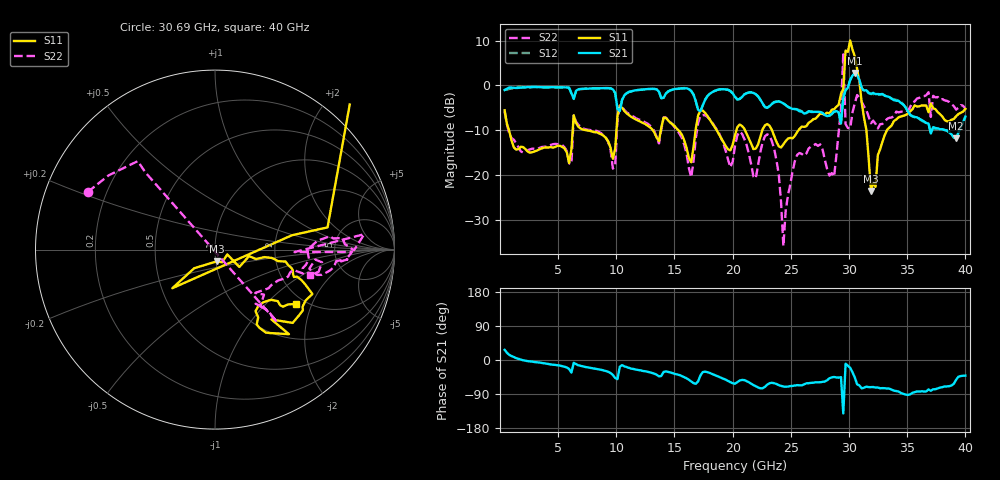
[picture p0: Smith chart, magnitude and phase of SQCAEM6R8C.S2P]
! Network Analyzer HP8722ES.07.66: Jul 25, 2000 Serial No. US39175408
! 26 Oct 2004  15:42:35
! Frequency  S11  S21  S12  S22
# HZ  S  DB R  50
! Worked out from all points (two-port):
!   201 points, 400 MHz to 40 GHz, reference 50 ohm
!   highest |S21| = 2.74 dB at 30.5 GHz (marker M1); lowest = -11.8 dB at 39.21 GHz (marker M2)
!   |S21| within 3 dB of the highest: 29.93 GHz to 31.05 GHz (1.12 GHz wide, 3.67 % of centre)
!   lowest |S11| = -23.6 dB at 31.88 GHz (marker M3), VSWR 1.14, Z = 50.6 - j6.64 ohm
!   |S11| at or under -10 dB: 771.5 MHz to 6.254 GHz (5.483 GHz wide, 156 % of centre); 7.361 GHz to 10.02 GHz (2.654 GHz wide, 30.6 % of centre); 23.38 GHz to 25.67 GHz (2.294 GHz wide, 9.35 % of centre)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
!   |S22| runs from -35.9 to 6.9 dB; largest |S21 - S12| = 0.17
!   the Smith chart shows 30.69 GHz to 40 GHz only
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4e8  -5.57 -66.2  -1.05 26.9  -1.00 30.4  -5.82 -58.9
7.132e9  -9.89 -101.3  -0.78 -17.1  -0.81 -17.5  -9.58 -112.5
1.3666e10  -12.44 -99.6  -1.43 -43.3  -1.44 -43.1  -12.98 -104.7
2.02e10  -11.18 -75.4  -2.60 -62.6  -2.54 -61.8  -13.53 -73.5
2.317e10  -9.04 -90.7  -4.67 -61.2  -4.63 -60.7  -11.22 -105.8
2.4358e10  -13.17 -70.4  -4.04 -70.1  -4.06 -69.2  -35.91 -91.4
2.5348e10  -11.27 -55.1  -5.31 -67.2  -5.27 -67.7  -16.91 -16.2
2.6932e10  -7.56 -54.4  -5.93 -59.9  -5.94 -59.7  -13.42 -31.8
2.8714e10  -5.36 -45.3  -5.89 -44.8  -5.84 -43.9  -20.38 20.9
2.9308e10  -1.94 -14.6  -8.52 -45.1  -8.47 -44.9  -5.33 25.2
2.9506e10  -0.79 7.4  -2.82 -141.1  -2.49 -127.9  6.91 45.4
2.9704e10  7.76 10.5  -1.11 -9.8  -0.94 -2.7  -8.66 -56.8
2.9902e10  7.48 -59.7  -0.52 -15.3  -0.47 -14.7  -9.53 9.0
3.01e10  10.01 -75.7  1.22 -20.4  1.15 -20.9  -9.62 16.1
3.0496e10  6.47 -104.7  2.74 -46.2  2.65 -46.1  -4.00 -7.8
3.0694e10  3.67 44.1  2.31 -64.1  2.25 -64.3  -2.17 155.7
3.1288e10  -7.22 10.5  -1.18 -73.2  -1.23 -73.2  -4.74 132.0
3.1486e10  -9.87 -137.9  -1.09 -70.3  -1.09 -69.1  -5.49 -49.4
3.1882e10  -23.59 -81.2  -1.90 -71.6  -1.96 -70.1  -8.47 -53.1
3.3466e10  -9.46 -9.2  -2.61 -75.4  -2.76 -75.5  -7.25 -20.3
3.9208e10  -6.90 -39.4  -11.83 -52.0  -11.70 -50.4  -5.42 -11.5
4e10  -5.27 -33.8  -6.98 -41.1  -7.13 -40.2  -5.20 -14.9
